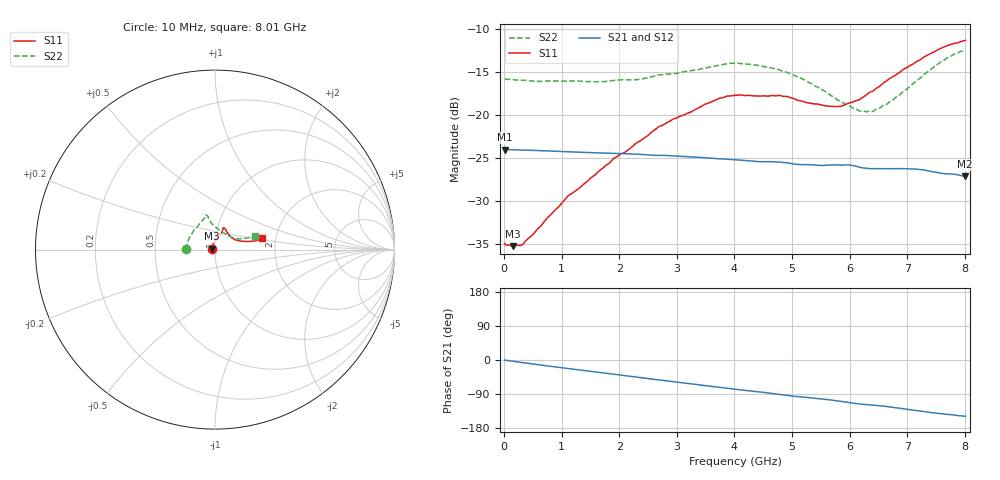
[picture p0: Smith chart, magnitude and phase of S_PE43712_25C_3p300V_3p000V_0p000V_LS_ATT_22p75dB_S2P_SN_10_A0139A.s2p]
! DEVICE ID: PE43712
! File Path: z:\PE43713\PE43713_CHAR_NOM_04292014\AMB\3p300\LS_ATT_22p75dB\PE43713_AMB_3p300V_3p000V_0p000V_LS_ATT_22p75dB_S2P_SN_10_A0139A.s2p
! Serial: 10
! Lot: A0139A
! Temp: 25C
! VDD: 3.300
! VSS: 0.000
! Control_Hi: 3.000
! Control_Lo: 0.000
! Attenuation Step: 22.75dB
! Port 1: RF1
! Port 2: RF2
! ThroughPath:1-2
! IDD: 0.0001469712
! ISS: -1.843e-007
#  Hz  S  RI  R  50
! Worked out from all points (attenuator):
!   801 points, 10 MHz to 8.01 GHz, reference 50 ohm
!   highest |S21| = -24.00 dB at 10 MHz (marker M1); lowest = -27.1 dB at 8 GHz (marker M2)
!   lowest |S11| = -35.2 dB at 160 MHz (marker M3), VSWR 1.04, Z = 48.4 + j0.522 ohm
!   |S11| at or under -10 dB: start of sweep to end of sweep
!   |S22| runs from -19.6 to -12.5 dB; largest |S21 - S12| = 0.00024
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1e7  -0.018 0.000684  0.0631 -0.00028  0.0631 -0.00029  -0.1623 0.00108
1.6e8  -0.0165 0.0054  0.0628 -0.0038  0.0628 -0.0038  -0.1601 0.0113
3.3e8  -0.015 0.00969  0.0622 -0.00768  0.0621 -0.00762  -0.1577 0.0206
1.11e9  -0.01 0.0324  0.0565 -0.0234  0.0565 -0.0234  -0.1434 0.065
1.35e9  -0.00638 0.0383  0.0542 -0.0276  0.0542 -0.0277  -0.137 0.0765
1.91e9  0.0051 0.0559  0.0475 -0.0366  0.0475 -0.0365  -0.1171 0.1077
2.28e9  0.0155 0.0663  0.0421 -0.0418  0.0421 -0.0417  -0.1015 0.1241
2.68e9  0.0272 0.0809  0.0358 -0.046  0.0358 -0.046  -0.0829 0.1495
3.71e9  0.0448 0.1156  0.0177 -0.0529  0.0176 -0.0529  -0.0546 0.1861
4.01e9  0.0473 0.1214  0.0123 -0.0537  0.0124 -0.0536  -0.0528 0.193
4.76e9  0.0542 0.1182  -0.000389 -0.0533  -0.000341 -0.0534  -0.0373 0.1801
5.12e9  0.0631 0.1037  -0.006 -0.0513  -0.00599 -0.0513  -0.029 0.1634
5.35e9  0.0685 0.0944  -0.00924 -0.0505  -0.00924 -0.0505  -0.0221 0.1497
5.82e9  0.0875 0.0701  -0.0163 -0.0486  -0.0162 -0.0486  0.00931 0.1204
6.18e9  0.1103 0.0555  -0.022 -0.0446  -0.0219 -0.0446  0.043 0.0962
6.4e9  0.1277 0.0512  -0.0236 -0.0427  -0.0235 -0.0427  0.0662 0.0815
6.68e9  0.155 0.0465  -0.0269 -0.0407  -0.0269 -0.0407  0.0976 0.0671
7.17e9  0.1998 0.0462  -0.0334 -0.0352  -0.0333 -0.0352  0.147 0.061
7.55e9  0.2356 0.0518  -0.0359 -0.029  -0.0358 -0.029  0.1883 0.067
7.81e9  0.2537 0.058  -0.0373 -0.0259  -0.0372 -0.0259  0.2126 0.0744
8e9  0.2633 0.0626  -0.0375 -0.0232  -0.0374 -0.0232  0.2227 0.0765
8.01e9  0.2638 0.0633  -0.0375 -0.0232  -0.0374 -0.0232  0.2233 0.0765
